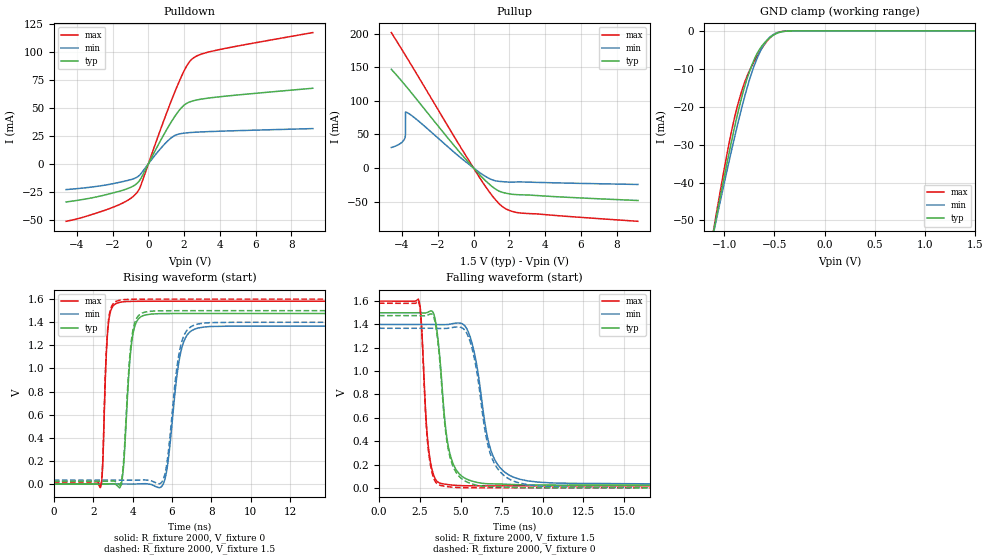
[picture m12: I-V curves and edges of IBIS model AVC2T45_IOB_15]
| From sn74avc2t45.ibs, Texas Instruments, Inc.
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[Model]   AVC2T45_IOB_15
Model_type  I/O
Vinl=0.49
Vinh=1.04
Enable   Active-High
Vref =   0
Rref =   2000
Cref =   15p
Vmeas =   0.75
| variable   typ   min   max
C_comp   5.16pF   4.56pF   5.78pF
| C_pullup   5.11pF   3.65pF   7.54pF
| C_pulldown   4.79pF   4.27pF   5.47pF
| C_tri-state   5.16pF   4.56pF   5.78pF
[Temperature Range]   40   100   -40
| Ambient temperature   25   85   -40
[Voltage range]   1.5   1.4   1.6
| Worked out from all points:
|   slope of the pulldown table from 0 to 0.225 V, typ, clamps not added: 32.1 ohm
|   slope of the pullup table from 0 to 0.225 V, typ, clamps not added: 33.9 ohm
|   GND clamp passes 1 mA (typ) near -0.50 V on its own axis
|   rising waveform, R_fixture 2000, V_fixture 0: 20-80 % time 328ps typ, 535ps min, 199ps max; typ from 0 V to 1.48 V
|   falling waveform, R_fixture 2000, V_fixture 1.5: 20-80 % time 632ps typ, 1.01ns min, 390ps max; typ from 1.5 V to 0.023 V
|   rising waveform, R_fixture 2000, V_fixture 1.5: 20-80 % time 325ps typ, 523ps min, 197ps max; typ from 0.023 V to 1.5 V
|   falling waveform, R_fixture 2000, V_fixture 0: 20-80 % time 633ps typ, 1ns min, 383ps max; typ from 1.48 V to 0 V
[GND Clamp]
| AVC2T45_IOB_15
|   Voltage   I(typ)   I(min)   I(max)
-4.6V     -597.8mA   -546.6mA   -662.5mA
-1.1V     -52.11mA   -52.52mA   -51.59mA
-1.075V   -48.66mA   -49.4mA    -47.7mA
-930mV    -29.5mA    -31.88mA   -26.82mA
-830mV    -17.94mA   -20.74mA   -16.24mA
-765mV    -12.02mA   -14.35mA   -11.48mA
-685mV    -6.644mA   -8.056mA   -7.261mA
-605mV    -3.35mA    -3.664mA   -3.806mA
-535mV    -1.602mA   -1.422mA   -1.608mA
-460mV    -500.6uA   -413.1uA   -383.6uA
-350mV    -38.76uA   -40.58uA   -15.38uA
1.5V      804.7pA    34.55nA    79.67pA
[Pulldown]
| AVC2T45_IOB_15A
|   Voltage   I(typ)   I(min)   I(max)
-4.6V     -34.07mA   -23.01mA   -51.35mA
-1.885V   -25.62mA   -17.44mA   -38.24mA
-1.09V    -21.68mA   -14.59mA   -31.97mA
-630mV    -17.39mA   -11.88mA   -25.55mA
-415mV    -12.94mA   -8.777mA   -18.95mA
595mV     18.22mA    11.97mA    26.91mA
1.265V    37.01mA    23.01mA    55.56mA
1.7V      47.29mA    26.56mA    72.61mA
2.03V     52.78mA    27.45mA    84.03mA
2.5V      56.24mA    28.09mA    94.31mA
3.84V     59.63mA    29.04mA    101.6mA
9.2V      67.51mA    31.46mA    117.2mA
[Pullup]
| AVC2T45_IOB_15A
|   Voltage   I(typ)   I(min)   I(max)
-4.6V     146.8mA    30.47mA    201.5mA
-4.1V     131.8mA    36.24mA    180.2mA
-3.85V    123.9mA    43.97mA    169.4mA
-3.81V    122.6mA    49.37mA    167.6mA
-3.805V   122.5mA    83.3mA     167.4mA
-3.785V   121.8mA    83.17mA    166.5mA
-3.155V   101.3mA    71.56mA    138.8mA
175mV     -5.197mA   -3.574mA   -7.497mA
980mV     -26.35mA   -16.94mA   -39.04mA
1.625V    -36.35mA   -20.39mA   -57.65mA
2.595V    -39.89mA   -20.78mA   -66.9mA
9.2V      -48.41mA   -24.54mA   -79.36mA
[Ramp]
| AVC2T45_IOB_15A
| variable   typ   min   max
dV/dt_r   0.91/3.42E-10   0.84/5.50E-10   0.97/2.05E-10
dV/dt_f   0.89/6.40E-10   0.83/1.01E-09   0.96/3.95E-10
R_load = 2000
[Rising Waveform]
| AVC2T45_IOB_15A
R_fixture =   2000
C_fixture =   0
L_fixture =   0
V_fixture =   0
V_fixture_min = 0
V_fixture_max = 0
|   Time   V(typ)   V(min)   V(max)
0s        19.4nV     97.73nV    508.8pV
2.385ns   26.23uV    1.704uV    -24.32mV
2.77ns    -39.44uV   -12.3uV    1.377V
3.33ns    -31.75mV   11.08uV    1.572V
3.99ns    1.266V     -139.7uV   1.581V
4.665ns   1.464V     2.716mV    1.582V
5.61ns    1.475V     21.79mV    1.582V
6.445ns   1.475V     1.136V     1.582V
7.345ns   1.475V     1.35V      1.582V
40ns      1.476V     1.367V     1.582V
[Falling Waveform]
| AVC2T45_IOB_15A
R_fixture =   2000
C_fixture =   0
L_fixture =   0
V_fixture =   1.5
V_fixture_min = 1.4
V_fixture_max = 1.6
|   Time   V(typ)   V(min)   V(max)
0s        1.5V       1.4V       1.6V
2.435ns   1.5V       1.4V       1.607V
3.03ns    1.508V     1.4V       337.9mV
3.77ns    1.035V     1.398V     39.01mV
4.18ns    403.1mV    1.399V     28.99mV
4.755ns   147.3mV    1.412V     21.05mV
5.685ns   58.2mV     1.241V     17.61mV
6.94ns    34.28mV    284.1mV    17.23mV
8.595ns   26.67mV    74.17mV    17.19mV
40ns      23.49mV    32.45mV    17.19mV
[Rising Waveform]
| AVC2T45_IOB_15A
R_fixture =   2000
C_fixture =   0
L_fixture =   0
V_fixture =   1.5
V_fixture_min = 1.4
V_fixture_max = 1.6
|   Time   V(typ)   V(min)   V(max)
0s        23.49mV    32.45mV    17.19mV
2.385ns   23.52mV    32.45mV    -6.653mV
2.75ns    23.37mV    32.44mV    1.368V
3.345ns   -9.339mV   32.46mV    1.591V
3.98ns    1.29V      32.32mV    1.599V
4.625ns   1.488V     35.01mV    1.6V
5.59ns    1.499V     51.96mV    1.6V
6.42ns    1.5V       1.176V     1.6V
7.315ns   1.5V       1.384V     1.6V
40ns      1.5V       1.4V       1.6V
[Falling Waveform]
| AVC2T45_IOB_15A
R_fixture =   2000
C_fixture =   0
L_fixture =   0
V_fixture =   0
V_fixture_min = 0
V_fixture_max = 0
|   Time   V(typ)   V(min)   V(max)
0s        1.476V     1.367V     1.582V
2.435ns   1.476V     1.367V     1.589V
3.03ns    1.483V     1.367V     311.9mV
3.75ns    1.036V     1.365V     21.4mV
4.165ns   388.3mV    1.367V     11.1mV
4.735ns   128.2mV    1.378V     3.527mV
5.665ns   34.78mV    1.209V     380.3uV
6.91ns    10.73mV    253.5mV    39uV
8.59ns    2.837mV    41.53mV    7.149uV
40ns      65.13nV    633.6nV    57.57nV
